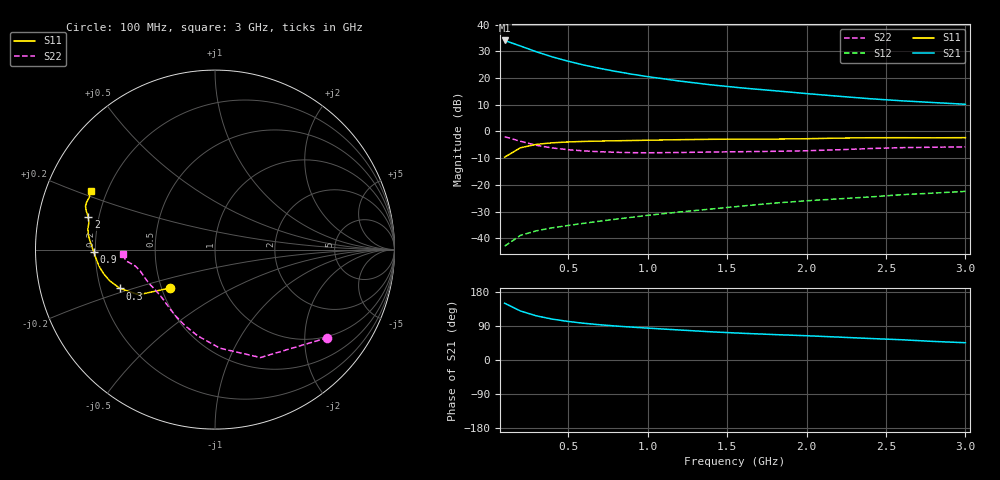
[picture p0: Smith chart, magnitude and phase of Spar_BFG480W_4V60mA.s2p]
! Filename: 460BFG480.001
! Title: BFG480W
! Bias: Vce=4V; Ic=60mA
! Company: NXP Semiconductors NL
! User: Quality&Reliability T&D
! Measure time: 10 Nov 1999 / 12:03:11
#  MHz  S  MA  R 50
! Freq  S11  S21  S12  S22  :
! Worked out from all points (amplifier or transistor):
!   20 points, 100 MHz to 3 GHz, reference 50 ohm
!   highest |S21| = 34.0 dB at 100 MHz (marker M1)
!   |S21| within 3 dB of that: start of sweep to 242.6 MHz
!   unconditionally stable (mu >= 1): 886.8 MHz to end of sweep
!   at 400 MHz: K = 0.69, MSG = 32.0 dB, |S12| = -36.1 dB
!   at 1.2 GHz: K = 1.06, MAG = 23.0 dB, |S12| = -30.2 dB
!   at 3 GHz: K = 1.05, MAG = 14.9 dB, |S12| = -22.4 dB
!   S11 on the Smith chart (normalised r, x): 100 MHz: 0.55, -0.27; 300 MHz: 0.28, -0.18; 900 MHz: 0.19, -0.01; 2 GHz: 0.16, +0.12; 3 GHz: 0.14, +0.22
100  0.3298 -139.5  50.38 149.8  0.007111 67.4  0.796 -38.1
200  0.4941 -149.4  39.64 129.3  0.01135 57.5  0.6525 -67.2
300  0.5721 -157.8  30.93 116.5  0.01379 54.7  0.55 -87.1
400  0.6119 -163.5  24.83 107.9  0.01568 55.0  0.49 -101.4
500  0.6351 -167.8  20.57 101.7  0.01736 56.5  0.454 -112.0
600  0.6496 -171.2  17.44 96.8  0.01908 58.2  0.4315 -120.0
700  0.6593 -174.0  15.1 93.0  0.02088 60.4  0.4163 -126.3
800  0.6675 -176.5  13.27 89.6  0.02277 62.4  0.4064 -131.6
900  0.6754 -178.8  11.79 86.8  0.02469 64.5  0.4004 -136.1
1000  0.6838 179.2  10.61 84.1  0.02683 66.0  0.3983 -140.3
1200  0.6997 175.8  8.77 79.2  0.03103 68.4  0.4027 -147.0
1400  0.7117 173.2  7.433 74.4  0.03525 70.0  0.4115 -152.0
1600  0.7176 170.7  6.485 70.5  0.04022 71.5  0.4173 -155.8
1800  0.7184 167.9  5.766 67.0  0.04559 72.6  0.4238 -159.8
2000  0.7292 165.6  5.105 64.0  0.05031 73.7  0.4341 -164.3
2200  0.749 163.3  4.557 60.5  0.05457 73.9  0.4531 -168.3
2400  0.7612 161.4  4.088 56.8  0.05937 73.7  0.4776 -170.9
2600  0.7625 159.8  3.737 53.4  0.06536 73.3  0.4967 -172.5
2800  0.7589 157.5  3.468 49.0  0.07008 72.1  0.5058 -174.4
3000  0.7638 154.8  3.219 45.6  0.07543 71.6  0.5133 -177.4
